PROGRAM p08_counter
VAR
	counter: CTUD;
	S0: BOOL;
	S1: BOOL;
	S2: BOOL;
	S3: BOOL;
	value: WORD;
END_VAR

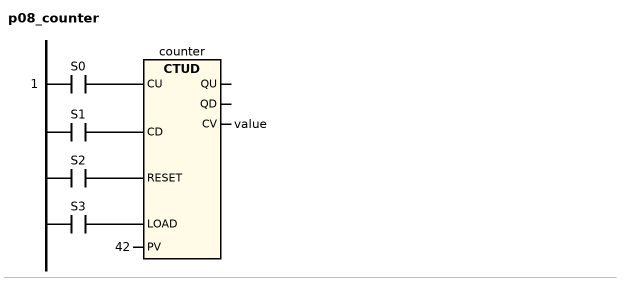
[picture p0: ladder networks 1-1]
// NETWORK 1
counter(CU := S0, CD := S1, RESET := S2, LOAD := S3, PV := 42, CV => value); // CTUD

END_PROGRAM
